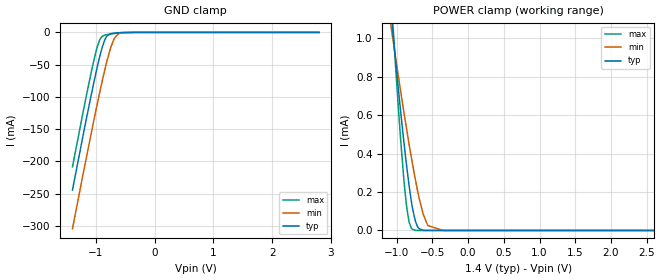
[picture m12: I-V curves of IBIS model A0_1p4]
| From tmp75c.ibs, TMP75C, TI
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|   Model
[Model]   A0_1p4
Model_type   Input
Vinl = 0.5
Vinh = 1.3
|   typ   min   max
C_comp   0.383pF   0.370pF   0.391pF
[Voltage Range]   1.4   1.39   1.41
[Temperature Range]   25   125   -40
[Power Clamp Reference]   1.4   1.39   1.41
[GND Clamp Reference]   0   0   0
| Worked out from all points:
|   GND clamp passes 1 mA (typ) near -0.68 V on its own axis
|   POWER clamp passes 1 mA (typ) near -1.05 V on its own axis
[GND Clamp]
|   Voltage   I(typ)   I(min)   I(max)
-1.4V     -244.5mA   -304.5mA   -208.6mA
-1.161V   -132.8mA   -192.7mA   -96.94mA
-1.035V   -77.01mA   -135.8mA   -42.95mA
-975.8mV  -52.72mA   -110mA     -21.86mA
-929.6mV  -35.18mA   -90.33mA   -10.36mA
-858.2mV  -13.47mA   -61.35mA   -4.448mA
-828.8mV  -7.788mA   -50.17mA   -3.769mA
-744.8mV  -1.881mA   -22.37mA   -2.431mA
-690.2mV  -1.069mA   -9.814mA   -1.697mA
-627.2mV  -552.2uA   -2.668mA   -977.9uA
-350mV    -14.71uA   -14.54uA   -26.47uA
2.8V      0A         0A         0A
[POWER Clamp]
|   Voltage   I(typ)   I(min)   I(max)
-1.4V     2.473mA    1.906mA    3.302mA
-1.182V   1.548mA    1.324mA    1.867mA
-1.047V   1.006mA    977.7uA    1.037mA
-946.4mV  624.9uA    727.9uA    480.7uA
-887.6mV  420.9uA    587.9uA    216.2uA
-828.8mV  239.8uA    453.6uA    48.31uA
-778.4mV  115uA      344.8uA    5.775uA
-702.8mV  16.59uA    197.5uA    140.1nA
-631.4mV  1.225uA    87.27uA    246.3pA
-564.2mV  89.04nA    25.53uA    0A
-350mV    0A         70.85nA    0A
2.8V      0A         0A         0A
